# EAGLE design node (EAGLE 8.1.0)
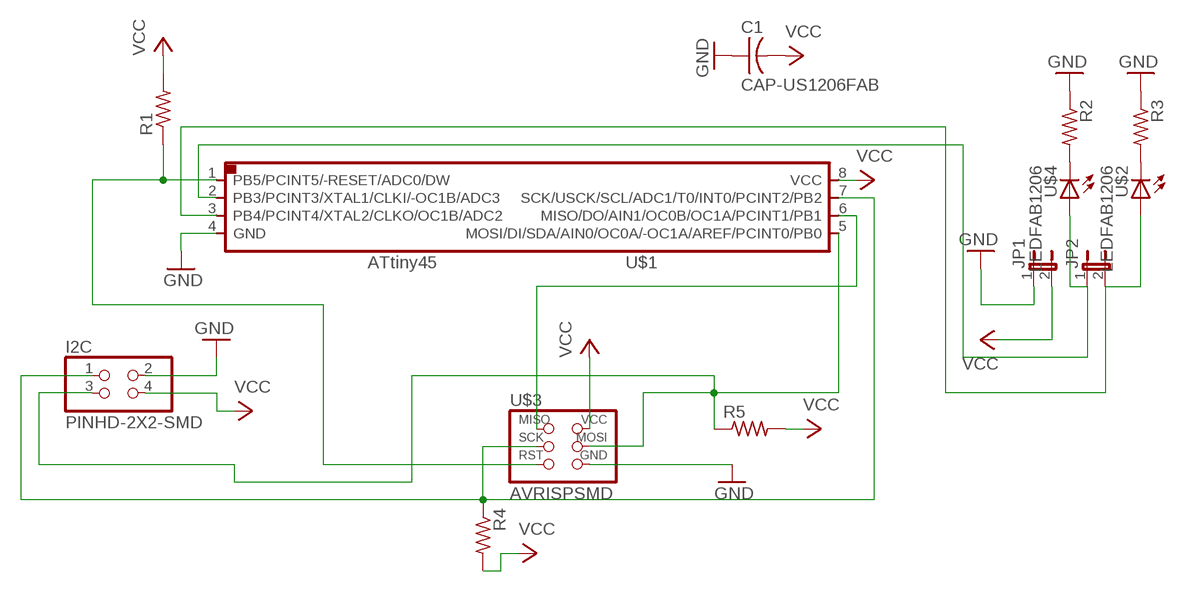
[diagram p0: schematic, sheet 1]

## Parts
C1  CAP-US1206FAB  [C1206FAB]
I2C  PINHD-2X2-SMD  [2X02SMD]
JP1  JP1E  [JP1]
JP2  JP1E  [JP1]
R1  RES-US1206FAB  [R1206FAB]
R2  RES-US1206FAB  [R1206FAB]
R3  RES-US1206FAB  [R1206FAB]
R4  RES-US1206FAB  [R1206FAB]
R5  RES-US1206FAB  [R1206FAB]
U$1  ATTINY45SI  [SOIC8]
U$2  LEDFAB1206  [LED1206FAB]
U$3  AVRISPSMD  [2X03SMD]
U$4  LEDFAB1206  [LED1206FAB]

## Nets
GND: C1.1 I2C.2 JP1.1 R2.1 R3.1 U$1.4(GND) U$3.6(GND)
N$1: R1.1 U$1.1(PB5/PCINT5/-RESET/ADC0/DW) U$3.5(RST)
N$2: U$1.6(MISO/DO/AIN1/OC0B/OC1A/PCINT1/PB1) U$3.1(MISO)
N$3: I2C.3 R5.1 U$1.5(MOSI/DI/SDA/AIN0/OC0A/-OC1A/AREF/PCINT0/PB0) U$3.4(MOSI)
N$4: I2C.1 R4.1 U$1.7(SCK/USCK/SCL/ADC1/T0/INT0/PCINT2/PB2) U$3.3(SCK)
N$5: R2.2 U$4.2(C)
N$6: R3.2 U$2.2(C)
N$7: JP2.2 U$1.3(PB4/PCINT4/XTAL2/CLKO/OC1B/ADC2) U$2.1(A)
N$9: JP2.1 U$1.2(PB3/PCINT3/XTAL1/CLKI/-OC1B/ADC3) U$4.1(A)
VCC: C1.2 I2C.4 JP1.2 R1.2 R4.2 R5.2 U$1.8(VCC) U$3.2(VCC)

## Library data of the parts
C1 = fab:CAP-US
I2C = fab:PINHD-2X2-SMD
JP1 JP2 = jumper:JP1E: JUMPER
R1-R5 = fab:RES-US: Resistor (US Symbol)
U$1 = fab:ATTINY45
U$2 U$4 = fab:LED: LED
U$3 = fab:AVRISP

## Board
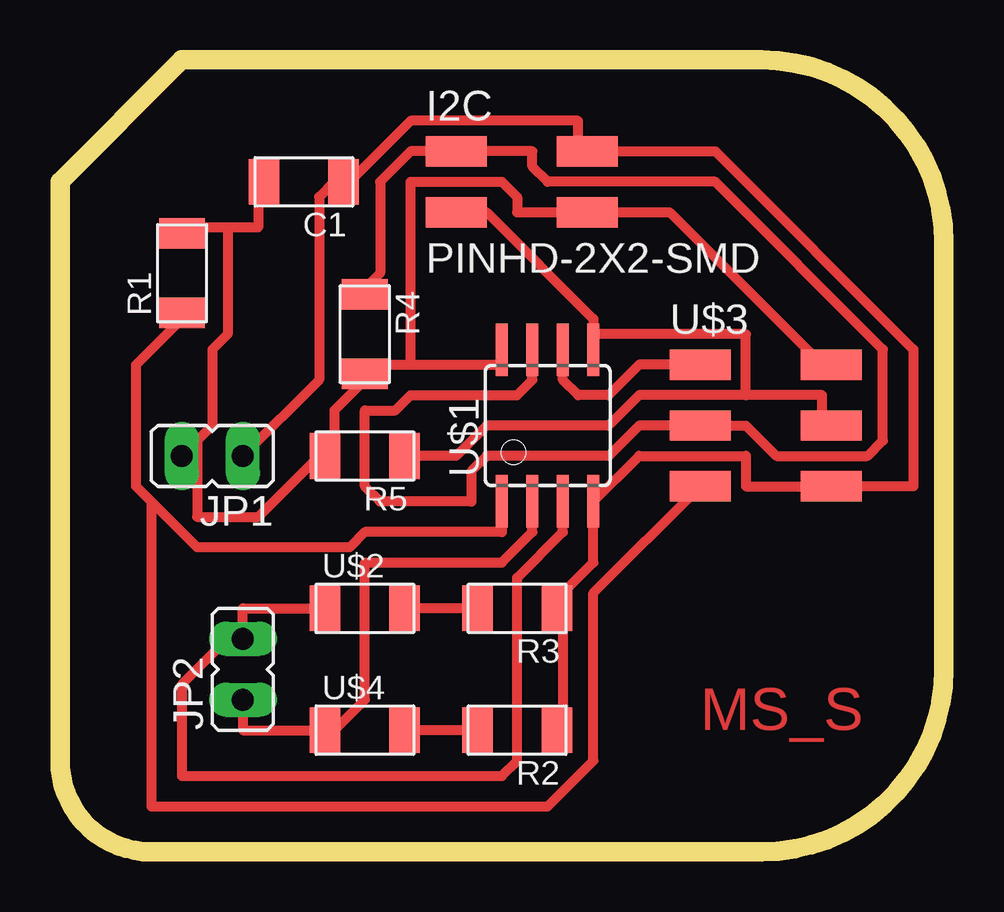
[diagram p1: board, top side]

Size 36.83 x 33.02 mm. Coordinates in mm from the lower left corner, seen from the top.
Outline: 29.21,33.02 arc-90 36.83,25.4 36.83,7.62 arc-90 29.21,0 3.81,0 arc-90 0,3.81 0,27.94 5.08,33.02 29.21,33.02
Copper layers (1*16): Top 0.035mm / dielectric 1.5mm / Bottom 0.035mm
Design rules "default *": minimum track width 16mil, minimum drill 24mil, track to track 16mil, track to pad 16mil, pad to pad 16mil, via to via 16mil, smd to smd 8mil, copper to edge 40mil, drill to drill 8mil, minimum pad ring 10mil, minimum via ring 8mil, stop-mask expansion 4mil, vias tented up to drill 0mil, thermal gap 10mil

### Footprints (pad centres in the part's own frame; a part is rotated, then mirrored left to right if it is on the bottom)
C1206FAB = smd 1.27 x 1.905: 1 -1.651,0; 2 1.651,0
2X02SMD = smd 2.54 x 1.27: 1 -2.54,1.27; 2 2.92,1.27; 3 -2.54,-1.27; 4 2.92,-1.27
JP1 = drill 0.914 long: 1 0,-1.27; 2 0,1.27
R1206FAB = smd 1.27 x 1.905: 1 -1.651,0; 2 1.651,0
SOIC8 = smd 0.5 x 2.2: 1 -1.905,-3.154; 2 -0.645,-3.154; 3 0.625,-3.154; 4 1.895,-3.154; 5 1.905,3.154; 6 0.635,3.154; 7 -0.635,3.154; 8 -1.905,3.154
LED1206FAB = smd 1.27 x 1.905: 1 -1.651,0; 2 1.651,0
2X03SMD = smd 2.54 x 1.27: 1 -2.54,2.54; 2 2.92,2.54; 3 -2.54,0; 4 2.92,0; 5 -2.54,-2.54; 6 2.92,-2.54

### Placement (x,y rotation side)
C1  10.16,27.94 180 top
I2C  19.05,27.94 0 top
JP1  6.35,16.51 90 top
JP2  7.62,7.62 0 top
R1  5.08,24.13 90 top
R2  19.05,5.08 180 top
R3  19.05,10.16 180 top
R4  12.7,21.59 270 top
R5  12.7,16.51 180 top
U$1  20.32,17.78 0 top
U$2  12.7,10.16 0 top
U$3  29.21,17.78 0 top
U$4  12.7,5.08 0 top

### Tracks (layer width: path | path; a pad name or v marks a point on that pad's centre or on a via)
GND
  Top 0.406: 20.96,10.16 20.96,5.08 R2.1 | 22.22,14.6 22.22,12.06 20.96,10.8 20.96,10.16 | 20.96,10.16 R3.1 | 22.22,14.6 24.13,16.51 28.57,16.51 28.57,15.24 U$3.6 35.56,15.24 35.56,20.95 27.3,29.21 I2C.2 21.59,29.21 21.59,30.48 14.61,30.48 12.07,27.94 C1.1 11.43,27.94 10.79,27.3 10.79,19.69 JP1.1 | 22.22,14.6 U$1.4
N$1
  Top 0.406: 3.81,14.6 5.71,12.7 12.07,12.7 12.7,13.34 18.41,13.34 U$1.1 | 3.81,14.6 3.17,15.24 3.17,20.32 5.08,22.23 R1.1 | U$3.5 22.22,10.8 22.22,3.81 20.32,1.9 3.81,1.9 3.81,14.6
N$2
  Top 0.406: U$1.6 20.96,19.69 21.59,19.05 22.86,19.05 24.13,20.32 U$3.1
N$3
  Top 0.406: 22.22,21.59 22.22,22.23 17.78,26.67 I2C.3 | R5.1 16.51,16.51 17.78,17.78 22.86,17.78 24.13,19.05 28.57,19.05 | 28.57,19.05 31.75,19.05 31.75,17.78 U$3.4 | 22.22,21.59 28.57,21.59 28.57,19.05 | 22.22,21.59 U$1.5
N$4
  Top 0.406: R4.1 12.7,23.49 13.33,24.13 13.33,27.94 14.61,29.21 I2C.1 19.68,29.21 19.68,28.57 20.32,27.94 27.3,27.94 34.29,20.95 34.29,17.14 33.66,16.51 29.84,16.51 28.57,17.78 U$3.3 24.13,17.78 22.86,16.51 17.78,16.51 17.14,15.88 17.14,14.6 13.33,14.6 12.7,15.24 12.7,18.41 13.97,18.41 14.61,19.05 19.05,19.05 19.68,19.69 U$1.7
N$5
  Top 0.406: R2.2 U$4.2
N$6
  Top 0.406: R3.2 U$2.2
N$7
  Top 0.406: U$2.1 7.62,10.16 7.62,9.52 | 7.62,9.52 5.08,6.98 5.08,3.17 18.41,3.17 19.05,3.81 19.05,11.43 20.96,13.34 20.96,14.6 U$1.3 | 7.62,9.52 JP2.2
N$9
  Top 0.406: JP2.1 7.62,5.08 U$4.1 11.43,5.08 12.7,6.35 12.7,12.06 18.41,12.06 19.68,13.34 19.68,14.6 U$1.2
VCC
  Top 0.406: U$3.2 31.75,20.32 25.4,26.67 I2C.4 19.05,26.67 19.05,27.3 18.41,27.94 14.61,27.94 14.61,20.32 | 14.61,20.32 12.7,20.32 R4.2 12.7,19.69 11.43,18.41 11.43,16.51 R5.2 10.79,16.51 8.25,13.97 5.71,13.97 5.71,17.14 | 14.61,20.32 18.41,20.32 U$1.8 | 6.98,26.03 8.25,26.03 8.25,27.94 C1.2 | 6.98,26.03 5.08,26.03 R1.2 | 5.71,17.14 6.35,17.78 6.35,20.95 6.98,21.59 6.98,26.03 | 5.71,17.14 JP1.2

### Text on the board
Top: MS_S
